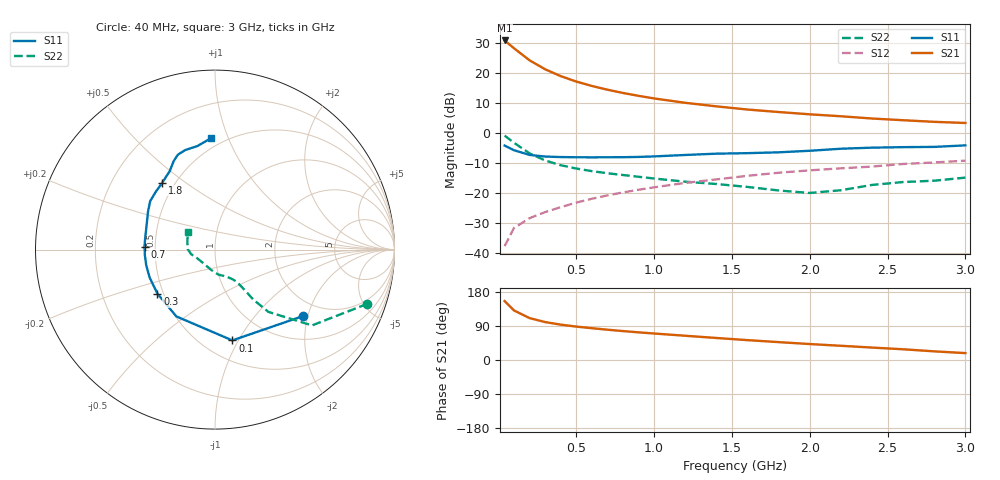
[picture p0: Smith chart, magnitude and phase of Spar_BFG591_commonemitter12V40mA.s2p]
! Filename:  BFG591D.S2P  Version:  4.0
! NXP part #: BFG591  Date: Jun 1994
! Bias condition: Vce=12V; Ic=40mA
#  MHz  S  MA  R  50
! Freq  S11  S21  S12  S22  !GUM [dB]
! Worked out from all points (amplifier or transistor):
!   21 points, 40 MHz to 3 GHz, reference 50 ohm
!   highest |S21| = 30.8 dB at 40 MHz (marker M1)
!   |S21| within 3 dB of that: start of sweep to 110.5 MHz
!   unconditionally stable (mu >= 1): 664.1 MHz to 2.188 GHz
!   at 300 MHz: K = 0.80, MSG = 23.8 dB, |S12| = -26.4 dB
!   at 1 GHz: K = 1.05, MAG = 13.4 dB, |S12| = -18.1 dB
!   at 3 GHz: K = 0.95, MSG = 6.3 dB, |S12| = -9.2 dB
!   S11 on the Smith chart (normalised r, x): 40 MHz: 1.57, -1.87; 100 MHz: 0.69, -0.94; 300 MHz: 0.46, -0.27; 700 MHz: 0.44, +0.01; 1.8 GHz: 0.43, +0.41; 3 GHz: 0.43, +0.87
40  0.615 -37.0  34.62 155.5  0.013 74.4  0.901 -19.6
100  0.515 -79.2  25.73 130.9  0.026 62.9  0.686 -38.0
200  0.43 -120.1  16.18 110.6  0.038 59.0  0.457 -49.4
300  0.404 -142.5  11.48 100.1  0.048 60.7  0.348 -52.6
400  0.396 -156.9  8.825 93.3  0.058 62.5  0.29 -53.5
500  0.393 -167.1  7.163 88.2  0.069 64.4  0.255 -54.4
600  0.392 -175.2  6.053 83.9  0.08 65.2  0.231 -55.4
700  0.393 177.9  5.241 80.0  0.091 65.9  0.213 -56.6
800  0.394 171.4  4.627 76.3  0.102 66.2  0.199 -58.3
900  0.398 165.2  4.142 73.0  0.113 66.4  0.186 -60.7
1000  0.406 159.6  3.748 69.9  0.124 66.3  0.174 -63.8
1200  0.429 150.4  3.171 64.0  0.147 65.3  0.154 -72.0
1400  0.451 143.2  2.767 58.1  0.168 63.7  0.141 -81.8
1600  0.46 136.4  2.45 52.4  0.193 62.8  0.126 -92.5
1800  0.475 128.2  2.226 47.2  0.217 59.9  0.11 -105.6
2000  0.504 120.1  2.04 42.1  0.238 58.3  0.1 -129.9
2200  0.545 114.9  1.892 37.5  0.257 56.2  0.111 -154.8
2400  0.568 111.3  1.736 32.8  0.275 55.3  0.136 -169.5
2600  0.579 106.6  1.626 28.3  0.304 51.8  0.152 178.8
2800  0.585 99.7  1.528 22.8  0.322 47.9  0.16 164.4
3000  0.62 92.2  1.463 18.2  0.345 46.5  0.18 147.2
